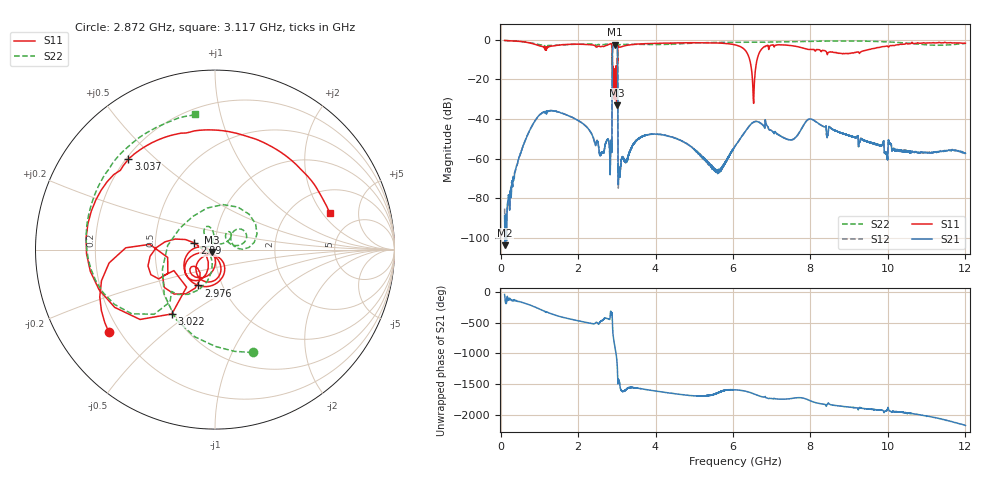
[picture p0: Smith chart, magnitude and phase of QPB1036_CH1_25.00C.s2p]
! TDS: K:\Engsetup\Winsaw\QPB1036_ALL
! Channel 1
! Ports=1 2
! seg 1=100.000000 1100.000000 101
! seg 2=1101.000000 1501.000000 401
! seg 3=1502.000000 2502.000000 101
! seg 4=2503.000000 3803.000000 1301
! seg 5=3804.000000 5004.000000 121
! seg 6=5005.000000 6005.000000 1001
! seg 7=6006.000000 8406.000000 241
! seg 8=8407.000000 10607.000000 2201
! seg 9=10608.000000 12008.000000 141
! Points=5609
! FailCode=0
! Topology=ALL_SE(12)
!VNA Cal loaded =QPB1036_ALL_25C
!PS1(V)= 5.000
!PS(mA)= 0.300
!PS2(V)= 0.630
!PS(mA)= -0.100
!PS3(V)= 0.630
!PS(mA)= 0.100
!PS4(V)= 1.170
!PS(mA)= -0.100
!Temp (C)= 25.00
# MHz S DB R 50
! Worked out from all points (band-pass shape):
!   5609 points, 100 MHz to 12.01 GHz, reference 50 ohm
!   highest |S21| = -2.41 dB at 2.955 GHz (marker M1); lowest = -103.9 dB at 110 MHz (marker M2)
!   |S21| within 3 dB of the highest: 2.889 GHz to 3.016 GHz (127.6 MHz wide, 4.32 % of centre)
!   lowest |S11| = -33.0 dB at 2.996 GHz (marker M3), VSWR 1.05, Z = 48.2 - j1.27 ohm
!   |S11| at or under -10 dB: 2.879456 GHz to 2.881392 GHz (1.936 MHz wide, 0.0672 % of centre); 2.886 GHz to 3.017 GHz (130.3 MHz wide, 4.41 % of centre); 6.433 GHz to 6.624 GHz (191.2 MHz wide, 2.93 % of centre)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
!   |S22| runs from -29.3 to -0.3 dB; largest |S21 - S12| = 0.0072
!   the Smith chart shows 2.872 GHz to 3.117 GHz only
!   S11 on the Smith chart (normalised r, x): 2.872 GHz: 0.16, -0.33; 2.89 GHz: 0.79, +0.06; 2.976 GHz: 0.77, -0.32; 3.022 GHz: 0.49, -0.43; 3.037 GHz: 0.21, +0.41; 3.117 GHz: 3.19, +2.37
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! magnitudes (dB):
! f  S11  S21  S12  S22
! 100 MHz  -0.3  -88.8  -85.3  -0.3
! 110 MHz  -0.3  -103.9  -97.7  -0.3
! 1.121 GHz  -4.0  -36.7  -36.7  -3.4
! 2.092 GHz  -2.2  -41.9  -41.9  -2.1
! 2.824 GHz  -2.1  -63.1  -62.9  -1.9
! 2.848 GHz  -1.9  -52.0  -52.2  -1.9
! 2.872 GHz  -2.5  -56.0  -56.0  -4.3
! 2.89 GHz  -18.4  -4.8  -4.8  -16.2
! 2.908 GHz  -17.0  -3.0  -3.0  -16.1
! 2.955 GHz  -29.4  -2.4  -2.4  -29.2
! 2.976 GHz  -13.1  -2.7  -2.7  -17.6
! 2.996 GHz  -33.0  -3.0  -3.0  -23.5
! 3.022 GHz  -7.3  -13.1  -13.1  -6.1
! 3.037 GHz  -3.1  -73.2  -72.4  -2.7
! 3.059 GHz  -3.6  -65.1  -64.9  -2.5
! 3.117 GHz  -3.5  -60.5  -60.6  -2.4
! 4.074 GHz  -1.7  -47.8  -47.7  -2.4
! 5.595 GHz  -1.6  -66.1  -66.4  -1.3
! 6.056 GHz  -2.5  -53.9  -53.7  -1.2
! 8.046 GHz  -4.8  -40.2  -40.2  -0.7
! 10.02 GHz  -3.6  -50.8  -50.7  -1.1
! 12.01 GHz  -1.7  -57.3  -57.2  -1.8
